| IBIS file stm32u375_385_ufbga64.ibs
[IBIS ver] 4.2
[File name] stm32u375_385_ufbga64.ibs
[File Rev] 1.2
[Date] 23-06-2025
[Source] Data Created at STMicroelectronics
[Notes]  File originated from ELDO simulations.
[Disclaimer]  This information is for modeling purpose only and is
   not guaranted. The information is subject to change without
   notice.
[Copyright] Copyright 2025 STMicroelectronics Inc.
|   Component stm32u375_385_ufbga64
[Component] stm32u375_385_ufbga64
[Manufacturer] STMicroelectronics
[Package]
| variable   typ   min   max
R_pkg  0  NA  NA
L_pkg  0  NA  NA
C_pkg  0  NA  NA
[Pin]   signal_name   model_name
A1  PC14-OSC32_IN  io_ft_tamp
A2  PC13  io8_ft_100m_v33
A3  PB9  io8_ft_100m_hslv
A4  PB4  io8_ft_100m_hslv
A5  PB3  io8_ft_100m_hslv
A6  PA15  io8_ft_100m
A7  PA14  io8_ft_100m
A8  PA13  io8_ft_100m
B1  PC15-OSC32_OUT  io_ft_tamp
B2  VBAT  power
B3  PB8  io8_ft_100m_hslv
B4  PH3-BOOT0  io8_ft_100m_hslv
B5  PD2  io8_ft_100m_hslv
B6  PC11  io8_ft_100m_hslv
B7  PC10  io8_ft_100m_hslv
B8  PA12  io8usb_ft_phy
C1  PH0-OSC_IN  io8_ft_100m
C2  VSS  gnd
C3  PB7  io8_ft_100m_hslv
C4  PB5  io8_ft_100m_hslv
C5  PC12  io8_ft_100m_hslv
C6  PA10  io8_ft_100m
C7  PA9  io8_ft_100m
C8  PA11  io8usb_ft_phy
D1  PH1-OSC_OUT  io8_ft_100m
D2  VDD  power
D3  PB6  io8_ft_100m_hslv
D4  VSS  gnd
D5  VSS  gnd
D6  VSS  gnd
D7  PA8  io8_ft_100m_hslv
D8  PC9  io8_ft_100m_hslv
E1  NRST  ioreset_v33
E2  PC1  io8_ft_100m_hslv
E3  PC0  io8_ft_100m_hslv
E4  VDD  power
E5  VDDUSB  power
E6  VDD  power
E7  PC7  io8_ft_100m_hslv
E8  PC8  io8_ft_100m_hslv
F1  VSSA  nc
F2  PC2  io8_ft_100m_hslv
F3  PA2  io8_ft_100m_hslv
F4  PA5  io8_ft_100m
F5  PB0  io8_ft_100m_hslv
F6  PC6  io8_ft_100m_hslv
F7  PB15  io8_ft_100m
F8  PB14  io8_ft_100m_hslv
G1  PC3  io8_ft_100m_hslv
G2  PA0  io8_ft_100m
G3  PA3  io8_ft_100m_hslv
G4  PA6  io8_ft_100m_hslv
G5  PB1  io8_ft_100m_hslv
G6  PB2  io8_ft_100m_hslv
G7  PB10  io8_ft_100m_hslv
G8  PB13  io8_ft_100m_hslv
H1  VDDA  nc
H2  PA1  io8_ft_100m_hslv
H3  PA4  io8_ft_100m_hslv
H4  PA7  io8_ft_100m_hslv
H5  PC4  io8_ft_100m_hslv
H6  PC5  io8_ft_100m
H7  VCAP  nc
H8  PB12  io8_ft_100m_hslv
[Package Model]   454-ufbga-5x5-64-ldo-250417
[Pin Mapping]   pulldown_ref   pullup_ref   | Comment
A1  gndio  vsw
A2  gndio  vsw
A3  gndio  vddio
A4  gndio  vddio
A5  gndio  vddio
A6  gndio  vddio
A7  gndio  vddio
A8  gndio  vddio
B1  gndio  vsw
B2  nc  vsw
B3  gndio  vddio
B4  gndio  vddio
B5  gndio  vddio
B6  gndio  vddio
B7  gndio  vddio
B8  gndio  vddusb  | Depending on IO usage
| B8  gndio  vddio  | Depending on IO usage
C1  gndio  vddio
C2  gndio  nc
C3  gndio  vddio
C4  gndio  vddio
C5  gndio  vddio
C6  gndio  vddio
C7  gndio  vddio
C8  gndio  vddusb  | Depending on IO usage
| C8  gndio  vddio  | Depending on IO usage
D1  gndio  vddio
D2  nc  vddio
D3  gndio  vddio
D4  gndio  nc
D5  gndio  nc
D6  gndio  nc
D7  gndio  vddio
D8  gndio  vddio
E1  gndio  vddio
E2  gndio  vddio
E3  gndio  vddio
E4  nc  vddio
E5  nc  vddusb
E6  nc  vddio
E7  gndio  vddio
E8  gndio  vddio
F1  nc  nc
F2  gndio  vddio
F3  gndio  vddio
F4  gndio  vddio
F5  gndio  vddio
F6  gndio  vddio
F7  gndio  vddio
F8  gndio  vddio
G1  gndio  vddio
G2  gndio  vddio
G3  gndio  vddio
G4  gndio  vddio
G5  gndio  vddio
G6  gndio  vddio
G7  gndio  vddio
G8  gndio  vddio
H1  nc  nc
H2  gndio  vddio
H3  gndio  vddio
H4  gndio  vddio
H5  gndio  vddio
H6  gndio  vddio
H7  nc  nc
H8  gndio  vddio
|[Diff Pin]  inv_pin  vdiff  tdelay_typ  tdelay_min  tdelay_max
|B8  C8  NA  NA  NA  NA
[Model Selector] io8_ft_100m
io8_ft_100m_ls_1v2  "GPIO 100MHz - 5V tolerant - low speed - 1.2V range"
io8_ft_100m_ls_1v8  "GPIO 100MHz - 5V tolerant - low speed - 1.8V range"
io8_ft_100m_ls_3v3  "GPIO 100MHz - 5V tolerant - low speed - 3.3V range"
io8_ft_100m_ms_1v2  "GPIO 100MHz - 5V tolerant - med speed - 1.2V range"
io8_ft_100m_ms_1v8  "GPIO 100MHz - 5V tolerant - med speed - 1.8V range"
io8_ft_100m_ms_3v3  "GPIO 100MHz - 5V tolerant - med speed - 3.3V range"
io8_ft_100m_fs_1v2  "GPIO 100MHz - 5V tolerant - fast speed - 1.2V range"
io8_ft_100m_fs_1v8  "GPIO 100MHz - 5V tolerant - fast speed - 1.8V range"
io8_ft_100m_fs_3v3  "GPIO 100MHz - 5V tolerant - fast speed - 3.3V range"
io8_ft_100m_hs_1v2  "GPIO 100MHz - 5V tolerant - high speed - 1.2V range"
io8_ft_100m_hs_1v8  "GPIO 100MHz - 5V tolerant - high speed - 1.8V range"
io8_ft_100m_hs_3v3  "GPIO 100MHz - 5V tolerant - high speed - 3.3V range"
[Model Selector] io8_ft_100m_hslv
io8_ft_100m_ls_1v2  "GPIO 100MHz - 5V tolerant - low speed - 1.2V range"
io8_ft_100m_ls_1v8  "GPIO 100MHz - 5V tolerant - low speed - 1.8V range"
io8_ft_100m_ls_3v3  "GPIO 100MHz - 5V tolerant - low speed - 3.3V range"
io8_ft_100m_ms_1v2  "GPIO 100MHz - 5V tolerant - med speed - 1.2V range"
io8_ft_100m_ms_1v8  "GPIO 100MHz - 5V tolerant - med speed - 1.8V range"
io8_ft_100m_ms_3v3  "GPIO 100MHz - 5V tolerant - med speed - 3.3V range"
io8_ft_100m_fs_1v2  "GPIO 100MHz - 5V tolerant - fast speed - 1.2V range"
io8_ft_100m_fs_1v8  "GPIO 100MHz - 5V tolerant - fast speed - 1.8V range"
io8_ft_100m_fs_3v3  "GPIO 100MHz - 5V tolerant - fast speed - 3.3V range"
io8_ft_100m_hs_1v2  "GPIO 100MHz - 5V tolerant - high speed - 1.2V range"
io8_ft_100m_hs_1v8  "GPIO 100MHz - 5V tolerant - high speed - 1.8V range"
io8_ft_100m_hs_3v3  "GPIO 100MHz - 5V tolerant - high speed - 3.3V range"
io8_ft_100m_hslv_ls_1v2  "GPIO 100MHz low voltage optimization - 5V tolerant - low speed - 1.2V range"
io8_ft_100m_hslv_ls_1v8  "GPIO 100MHz low voltage optimization - 5V tolerant - low speed - 1.8V range"
io8_ft_100m_hslv_ls_2v5  "GPIO 100MHz low voltage optimization - 5V tolerant - low speed - 3.3V range"
io8_ft_100m_hslv_ms_1v2  "GPIO 100MHz low voltage optimization - 5V tolerant - med speed - 1.2V range"
io8_ft_100m_hslv_ms_1v8  "GPIO 100MHz low voltage optimization - 5V tolerant - med speed - 1.8V range"
io8_ft_100m_hslv_ms_2v5  "GPIO 100MHz low voltage optimization - 5V tolerant - med speed - 3.3V range"
io8_ft_100m_hslv_fs_1v2  "GPIO 100MHz low voltage optimization - 5V tolerant - fast speed - 1.2V range"
io8_ft_100m_hslv_fs_1v8  "GPIO 100MHz low voltage optimization - 5V tolerant - fast speed - 1.8V range"
io8_ft_100m_hslv_fs_2v5  "GPIO 100MHz low voltage optimization - 5V tolerant - fast speed - 3.3V range"
io8_ft_100m_hslv_hs_1v2  "GPIO 100MHz low voltage optimization - 5V tolerant - high speed - 1.2V range"
io8_ft_100m_hslv_hs_1v8  "GPIO 100MHz low voltage optimization - 5V tolerant - high speed - 1.8V range"
io8_ft_100m_hslv_hs_2v5  "GPIO 100MHz low voltage optimization - 5V tolerant - high speed - 3.3V range"
[Model Selector] io8_ft_100m_v33
io8_ft_100m_v33_ls_1v2  "GPIO_V33 100MHz - 5V tolerant - low speed - 1.2V range"
io8_ft_100m_v33_ls_1v8  "GPIO_V33 100MHz - 5V tolerant - low speed - 1.8V range"
io8_ft_100m_v33_ls_3v3  "GPIO_V33 100MHz - 5V tolerant - low speed - 3.3V range"
io8_ft_100m_v33_ms_1v2  "GPIO_V33 100MHz - 5V tolerant - med speed - 1.2V range"
io8_ft_100m_v33_ms_1v8  "GPIO_V33 100MHz - 5V tolerant - med speed - 1.8V range"
io8_ft_100m_v33_ms_3v3  "GPIO_V33 100MHz - 5V tolerant - med speed - 3.3V range"
io8_ft_100m_v33_fs_1v2  "GPIO_V33 100MHz - 5V tolerant - fast speed - 1.2V range"
io8_ft_100m_v33_fs_1v8  "GPIO_V33 100MHz - 5V tolerant - fast speed - 1.8V range"
io8_ft_100m_v33_fs_3v3  "GPIO_V33 100MHz - 5V tolerant - fast speed - 3.3V range"
io8_ft_100m_v33_hs_1v2  "GPIO_V33 100MHz - 5V tolerant - high speed - 1.2V range"
io8_ft_100m_v33_hs_1v8  "GPIO_V33 100MHz - 5V tolerant - high speed - 1.8V range"
io8_ft_100m_v33_hs_3v3  "GPIO_V33 100MHz - 5V tolerant - high speed - 3.3V range"
[Model Selector] io8usb_ft_phy
io8_ft_100m_ls_1v2  "GPIO 100MHz - 5V tolerant - low speed - 1.2V range"
io8_ft_100m_ls_1v8  "GPIO 100MHz - 5V tolerant - low speed - 1.8V range"
io8_ft_100m_ls_3v3  "GPIO 100MHz - 5V tolerant - low speed - 3.3V range"
io8_ft_100m_ms_1v2  "GPIO 100MHz - 5V tolerant - med speed - 1.2V range"
io8_ft_100m_ms_1v8  "GPIO 100MHz - 5V tolerant - med speed - 1.8V range"
io8_ft_100m_ms_3v3  "GPIO 100MHz - 5V tolerant - med speed - 3.3V range"
io8_ft_100m_fs_1v2  "GPIO 100MHz - 5V tolerant - fast speed - 1.2V range"
io8_ft_100m_fs_1v8  "GPIO 100MHz - 5V tolerant - fast speed - 1.8V range"
io8_ft_100m_fs_3v3  "GPIO 100MHz - 5V tolerant - fast speed - 3.3V range"
io8_ft_100m_hs_1v2  "GPIO 100MHz - 5V tolerant - high speed - 1.2V range"
io8_ft_100m_hs_1v8  "GPIO 100MHz - 5V tolerant - high speed - 1.8V range"
io8_ft_100m_hs_3v3  "GPIO 100MHz - 5V tolerant - high speed - 3.3V range"
io8usb_ft_phy_hs_3v3   "USB full speed"
io8usb_ft_phy_ls_3v3   "USB low speed"
[Model Selector] io_ft_tamp
io_ft_tamp_ls_1v2 "io8_ft tamp low speed @ 1.2V"
io_ft_tamp_ls_1v8 "io8_ft tamp low speed @ 1.8V"
io_ft_tamp_ls_3v3 "io8_ft tamp low speed @ 3.3V"
io_ft_tamp_ms_1v2 "io8_ft tamp med speed @ 1.2V"
io_ft_tamp_ms_1v8 "io8_ft tamp med speed @ 1.8V"
io_ft_tamp_ms_3v3 "io8_ft tamp med speed @ 3.3V"
io_ft_tamp_fs_1v2 "io8_ft tamp fast speed @ 1.2V"
io_ft_tamp_fs_1v8 "io8_ft tamp fast speed @ 1.8V"
io_ft_tamp_fs_3v3 "io8_ft tamp fast speed @ 3.3V"
io_ft_tamp_hs_1v2 "io8_ft tamp high speed @ 1.2V"
io_ft_tamp_hs_1v8 "io8_ft tamp high speed @ 1.8V"
io_ft_tamp_hs_3v3 "io8_ft tamp high speed @ 3.3V"
[Model Selector] ioreset_v33
ioreset_v33_1v2 "Reset PAD. 5V tolerant. 1.2V range"
ioreset_v33_1v8 "Reset PAD. 5V tolerant. 1.8V range"
ioreset_v33_3v3 "Reset PAD. 5V tolerant. 3.3V range"
[Define Package Model]  454-ufbga-5x5-64-ldo-250417
[Manufacturer]  unknown
[OEM]  unknown
[Description]  unknown
[Number Of Pins]  59
[Pin Numbers]
| Pin Name Terminal   Net Name   Starting Node   Ending Node
E1 | NRST
G2 | PA0
H2 | PA1
F3 | PA2
G3 | PA3
H3 | PA4
F4 | PA5
G4 | PA6
H4 | PA7
D7 | PA8
C7 | PA9
C6 | PA10
C8 | PA11
B8 | PA12
A8 | PA13
A7 | PA14
A6 | PA15
F5 | PB0
G5 | PB1
G6 | PB2
A5 | PB3
A4 | PB4
C4 | PB5
D3 | PB6
C3 | PB7
B3 | PB8
A3 | PB9
G7 | PB10
H8 | PB12
G8 | PB13
F8 | PB14
F7 | PB15
E3 | PC0
E2 | PC1
F2 | PC2
G1 | PC3
H5 | PC4
H6 | PC5
F6 | PC6
E7 | PC7
E8 | PC8
D8 | PC9
B7 | PC10
B6 | PC11
C5 | PC12
A2 | PC13
A1 | PC14-OSC32_IN
B1 | PC15-OSC32_OUT
B5 | PD2
C1 | PH0-OSC_IN
D1 | PH1-OSC_OUT
B4 | PH3-BOOT0
B2 | VBAT
H7 | VCAP
D2 | VDD
H1 | VDDA
E5 | VDDUSB
C2 | VSS
F1 | VSSA
|[Merged Pins]  D2
|E4  |  VDD
|E6  |  VDD
|[Merged Pins]  C2
|D4  |  VSS
|D5  |  VSS
|D6  |  VSS
[Model Data]
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[End Model Data]
[End Package Model]
|End [Component]
| Models and submodels in the file (53): io8_ft_100m_fs_1v2 (I/O), io8_ft_100m_fs_1v8 (I/O), io8_ft_100m_fs_3v3 (I/O), io8_ft_100m_hs_1v2 (I/O), io8_ft_100m_hs_1v8 (I/O), io8_ft_100m_hs_3v3 (I/O), io8_ft_100m_hslv_fs_1v2 (I/O), io8_ft_100m_hslv_fs_1v8 (I/O), io8_ft_100m_hslv_fs_2v5 (I/O), io8_ft_100m_hslv_hs_1v2 (I/O), io8_ft_100m_hslv_hs_1v8 (I/O), io8_ft_100m_hslv_hs_2v5 (I/O), io8_ft_100m_hslv_ls_1v2 (I/O), io8_ft_100m_hslv_ls_1v8 (I/O), io8_ft_100m_hslv_ls_2v5 (I/O), io8_ft_100m_hslv_ms_1v2 (I/O), io8_ft_100m_hslv_ms_1v8 (I/O), io8_ft_100m_hslv_ms_2v5 (I/O), io8_ft_100m_ls_1v2 (I/O), io8_ft_100m_ls_1v8 (I/O), io8_ft_100m_ls_3v3 (I/O), io8_ft_100m_ms_1v2 (I/O), io8_ft_100m_ms_1v8 (I/O), io8_ft_100m_ms_3v3 (I/O), io8_ft_100m_v33_fs_1v2 (I/O), io8_ft_100m_v33_fs_1v8 (I/O), io8_ft_100m_v33_fs_3v3 (I/O), io8_ft_100m_v33_hs_1v2 (I/O), io8_ft_100m_v33_hs_1v8 (I/O), io8_ft_100m_v33_hs_3v3 (I/O), io8_ft_100m_v33_ls_1v2 (I/O), io8_ft_100m_v33_ls_1v8 (I/O), io8_ft_100m_v33_ls_3v3 (I/O), io8_ft_100m_v33_ms_1v2 (I/O), io8_ft_100m_v33_ms_1v8 (I/O), io8_ft_100m_v33_ms_3v3 (I/O), io8usb_ft_phy_hs_3v3 (I/O), io8usb_ft_phy_ls_3v3 (I/O), io_ft_tamp_fs_1v2 (I/O), io_ft_tamp_fs_1v8 (I/O), io_ft_tamp_fs_3v3 (I/O), io_ft_tamp_hs_1v2 (I/O), io_ft_tamp_hs_1v8 (I/O), io_ft_tamp_hs_3v3 (I/O), io_ft_tamp_ls_1v2 (I/O), io_ft_tamp_ls_1v8 (I/O), io_ft_tamp_ls_3v3 (I/O), io_ft_tamp_ms_1v2 (I/O), io_ft_tamp_ms_1v8 (I/O), io_ft_tamp_ms_3v3 (I/O), ioreset_v33_1v2 (I/O_open_drain), ioreset_v33_1v8 (I/O_open_drain), ioreset_v33_3v3 (I/O_open_drain)
